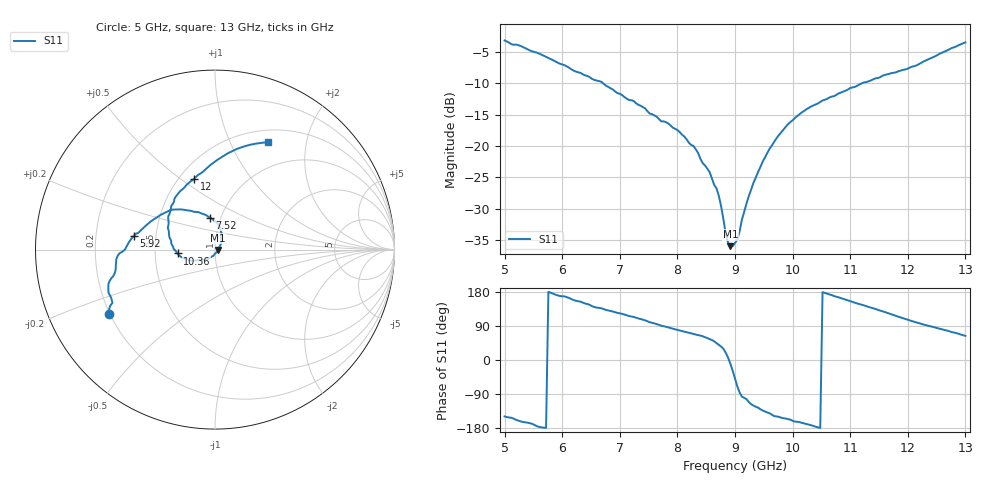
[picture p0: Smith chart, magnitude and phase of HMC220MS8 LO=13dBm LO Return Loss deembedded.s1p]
!Hittite Microwave Corporation
!12 Elizabeth Drive
!Chelmsford, MA 01824
!Tel: 978-250-3343
!Fax: 978-250-3373
!Device: HMC220MS8, 5-12 GHz, GaAS MMIC SMT Double-Balanced Mixer in 8-lead MSOP package
!Misc: LO power level=13dBm, Room
# MHZ S MA R 50
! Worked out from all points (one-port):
!   201 points, 5 GHz to 13 GHz, reference 50 ohm
!   lowest |S11| = -35.9 dB at 8.92 GHz (marker M1), VSWR 1.03, Z = 51.6 - j0.286 ohm
!   |S11| at or under -10 dB: 6.706 GHz to 11.21 GHz (4.504 GHz wide, 50.3 % of centre)
!   S11 on the Smith chart (normalised r, x): 5 GHz: 0.20, -0.27; 5.92 GHz: 0.37, +0.07; 7.52 GHz: 0.88, +0.33; 10.36 GHz: 0.65, -0.03; 12 GHz: 0.59, +0.57; 13 GHz: 0.65, +1.40
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5000  0.69 -148.8
5280  0.624 -162.1
5600  0.542 -176.5
5920  0.46 170.6
6000  0.445 168.2
6560  0.335 139.8
7000  0.26 123.2
7520  0.181 99.7
8000  0.134 79.5
8280  0.1 68.8
8560  0.062 54.9
8720  0.04 40.2
8840  0.02 19.0
8880  0.017 6.1
8920  0.016 -10.0
9000  0.017 -48.7
9040  0.018 -69.6
9120  0.026 -96.8
9240  0.04 -111.1
9480  0.075 -133.3
9760  0.122 -149.8
10000  0.16 -160.4
10360  0.21 -174.1
11000  0.289 155.4
11560  0.362 128.6
12000  0.412 106.2
12480  0.518 85.7
13000  0.666 63.7
